|-- THIS SOFTWARE IS PROVIDED BY FREESCALE "AS IS" AND ANY EXPRESSED OR
|-- IMPLIED WARRANTIES, INCLUDING, BUT NOT LIMITED TO, THE IMPLIED WARRANTIES
|-- OF MERCHANTABILITY AND FITNESS FOR A PARTICULAR PURPOSE ARE DISCLAIMED.
|-- IN NO EVENT SHALL FREESCALE OR ITS CONTRIBUTORS BE LIABLE FOR ANY DIRECT,
|-- INDIRECT, INCIDENTAL, SPECIAL, EXEMPLARY, OR CONSEQUENTIAL DAMAGES
|-- (INCLUDING, BUT NOT LIMITED TO, PROCUREMENT OF SUBSTITUTE GOODS OR
|-- SERVICES; LOSS OF USE, DATA, OR PROFITS; OR BUSINESS INTERRUPTION)
|-- HOWEVER CAUSED AND ON ANY THEORY OF LIABILITY, WHETHER IN CONTRACT,
|-- STRICT LIABILITY, OR TORT (INCLUDING NEGLIGENCE OR OTHERWISE) ARISING
|-- IN ANY WAY OUT OF THE USE OF THIS SOFTWARE, EVEN IF ADVISED OF
|-- THE POSSIBILITY OF SUCH DAMAGE.
[IBIS Ver]   5.0
[Comment Char] |_char
[File name]   k10_120_144lqfp_full.ibs
[File Rev]   1.2
[Date]   12/03/2013
[Source]   Freescale, MSG, MCD, Design
[Notes]   IBIS model for K10 microprocessor covers 1.71 - 3.6V range
[Disclaimer]   The model given below represents 144LQFP package on K10 family
[Copyright]   Copyright, Freescale, Inc., 2013
|  Component K10
[Component]   K10
[Manufacturer]  Freescale, Inc.
[Package]
|   typ   min   max
R_pkg   0.13889   0.089996   0.16304
L_pkg   6.188e-9   4.6e-9   7.753e-9
C_pkg   1.406e-12   1.199e-12   1.711e-12
[Pin]   Signal_name   model_name   R_pin   L_pin   C_pin
31   VDDA   POWER
5   VDD   POWER
16   VDD   POWER
43   VDD   POWER
56   VDD   POWER
70   VDD   POWER
94   VDD   POWER
108   VDD   POWER
122   VDD   POWER
135   VDD   POWER
42   VBAT   POWER
36   ADC0SE16   NC   0.14814   6.799e-9   1.29e-12
35   ADC1SE16   NC   0.15075   5.874e-9   1.605e-12
38   DAC0OUT   NC   0.1439   7.173e-9   1.633e-12
39   DAC1OUT   NC   0.14181   7.031e-9   1.609e-12
41   EXTAL32   NC   0.15225   6.57e-9   1.571e-12
28   PGA0DM   NC   0.12556   5.957e-9   1.439e-12
27   PGA0DP   NC   0.12328   5.956e-9   1.323e-12
30   PGA1DM   NC   0.13896   5.302e-9   1.498e-12
29   PGA1DP   NC   0.12975   5.793e-9   1.428e-12
24   PGA2DM   NC   0.12612   5.426e-9   1.253e-12
23   PGA2DP   NC   0.13132   5.164e-9   1.242e-12
26   PGA3DM   NC   0.12285   5.882e-9   1.338e-12
25   PGA3DP   NC   0.12278   5.637e-9   1.298e-12
50   PTA0   io_5vtol   0.14278   6.159e-9   1.422e-12
51   PTA1   io_5vtol   0.14286   6.108e-9   1.337e-12
52   PTA2   io_5vtol   0.14332   5.98e-9   1.337e-12
53   PTA3   io_5vtol   0.14456   5.799e-9   1.346e-12
54   PTA4   io_5vtol   0.14764   5.555e-9   1.299e-12
55   PTA5   io_5vtol   0.1539   5.005e-9   1.264e-12
58   PTA6   io_fast_5vtol  0.14954   5.263e-9   1.291e-12
59   PTA7   io_fast_5vtol  0.14483   5.816e-9   1.336e-12
60   PTA8   io_fast_5vtol  0.14374   6.082e-9   1.385e-12
61   PTA9   io_fast_5vtol  0.1435   6.256e-9   1.329e-12
62   PTA10   io_fast_5vtol  0.14504   6.55e-9   1.37e-12
63   PTA11   io_fast_5vtol  0.14604   6.721e-9   1.362e-12
64   PTA12   io_fast_5vtol  0.14817   6.838e-9   1.393e-12
65   PTA13   io_fast_5vtol  0.15098   6.974e-9   1.475e-12
66   PTA14   io_fast_5vtol  0.15439   7.067e-9   1.507e-12
67   PTA15   io_fast_5vtol  0.1589   7.1e-9   1.585e-12
68   PTA16   io_fast_5vtol  0.15577   6.721e-9   1.564e-12
69   PTA17   io_fast_5vtol  0.16419   6.271e-9   1.534e-12
72   PTA18   io_5vtol   0.16205   6.44e-9   1.293e-12
73   PTA19   io_5vtol   0.15246   7.525e-9   1.292e-12
75   PTA24   io_fast_5vtol  0.14705   7.251e-9   1.711e-12
76   PTA25   io_fast_5vtol  0.14202   7.111e-9   1.574e-12
77   PTA26   io_fast_5vtol  0.13768   6.963e-9   1.55e-12
78   PTA27   io_fast_5vtol  0.13385   6.813e-9   1.519e-12
79   PTA28   io_fast_5vtol  0.13044   6.629e-9   1.413e-12
80   PTA29   io_fast_5vtol  0.12785   6.516e-9   1.437e-12
81   PTB0   io_5vtol   0.12934   6.478e-9   1.329e-12
82   PTB1   io_5vtol   0.12678   6.332e-9   1.37e-12
83   PTB2   io_5vtol   0.12544   6.284e-9   1.394e-12
84   PTB3   io_5vtol   0.12339   6.065e-9   1.249e-12
85   PTB4   io_5vtol   0.12238   5.954e-9   1.26e-12
86   PTB5   io_5vtol   0.12176   5.806e-9   1.298e-12
87   PTB6   io_5vtol   0.12189   5.734e-9   1.29e-12
88   PTB7   io_5vtol   0.12236   5.627e-9   1.342e-12
89   PTB8   io_5vtol   0.12359   5.523e-9   1.305e-12
90   PTB9   io_5vtol   0.12579   5.377e-9   1.238e-12
91   PTB10   io_5vtol   0.12906   5.15e-9   1.278e-12
92   PTB11   io_5vtol   0.13573   4.6e-9   1.242e-12
95   PTB16   io_5vtol   0.13029   4.886e-9   1.199e-12
96   PTB17   io_5vtol   0.12755   5.429e-9   1.322e-12
97   PTB18   io_5vtol   0.12784   5.737e-9   1.313e-12
98   PTB19   io_5vtol   0.1267   6.027e-9   1.37e-12
99   PTB20   io_5vtol   0.12858   6.208e-9   1.359e-12
100   PTB21   io_5vtol   0.12421   6.241e-9   1.419e-12
101   PTB22   io_5vtol   0.12648   6.392e-9   1.422e-12
102   PTB23   io_5vtol   0.12927   6.504e-9   1.503e-12
103   PTC0   io_5vtol   0.13297   6.607e-9   1.602e-12
104   PTC1   io_5vtol   0.1375   6.627e-9   1.536e-12
105   PTC2   io_5vtol   0.14401   6.506e-9   1.577e-12
106   PTC3   io_5vtol   0.15452   5.98e-9   1.59e-12
109   PTC4   io_5vtol   0.15191   7.275e-9   1.253e-12
110   PTC5   io_5vtol   0.14762   7.211e-9   1.535e-12
111   PTC6   io_5vtol   0.14439   7.113e-9   1.542e-12
112   PTC7   io_5vtol   0.14253   7.08e-9   1.527e-12
113   PTC8   io_5vtol   0.14011   6.886e-9   1.414e-12
114   PTC9   io_5vtol   0.13988   6.924e-9   1.489e-12
115   PTC10   io_5vtol   0.13903   6.796e-9   1.48e-12
116   PTC11   io_5vtol   0.14399   6.78e-9   1.353e-12
117   PTC12   io_5vtol   0.14328   6.589e-9   1.442e-12
118   PTC13   io_5vtol   0.1433   6.308e-9   1.363e-12
119   PTC14   io_5vtol   0.14522   6.04e-9   1.387e-12
120   PTC15   io_5vtol   0.15252   5.309e-9   1.347e-12
123   PTC16   io_5vtol   0.15245   5.32e-9   1.261e-12
124   PTC17   io_5vtol   0.14692   5.762e-9   1.317e-12
125   PTC18   io_5vtol   0.14506   5.937e-9   1.38e-12
126   PTC19   io_5vtol   0.14439   6.01e-9   1.303e-12
127   PTD0   io_5vtol   0.14383   6.074e-9   1.304e-12
128   PTD1   io_5vtol   0.1432   6.11e-9   1.332e-12
129   PTD2   io_5vtol   0.14304   6.098e-9   1.298e-12
130   PTD3   io_5vtol   0.14369   6.113e-9   1.374e-12
131   PTD4   io_5vtol   0.14485   6.055e-9   1.311e-12
132   PTD5   io_5vtol   0.14745   5.946e-9   1.34e-12
133   PTD6   io_5vtol   0.15299   5.562e-9   1.278e-12
136   PTD7   io_5vtol   0.094519   5.239e-9   1.36e-12
137   PTD8   io_5vtol   0.14944   6.47e-9   1.472e-12
138   PTD9   io_5vtol   0.1483   6.789e-9   1.563e-12
139   PTD10   io_5vtol   0.14911   7.035e-9   1.591e-12
140   PTD11   io_5vtol   0.15067   7.248e-9   1.566e-12
141   PTD12   io_5vtol   0.14434   7.223e-9   1.472e-12
142   PTD13   io_5vtol   0.14611   7.405e-9   1.666e-12
143   PTD14   io_5vtol   0.14849   7.501e-9   1.697e-12
144   PTD15   io_5vtol   0.15161   7.753e-9   1.354e-12
1   PTE0   io_5vtol   0.14437   7.313e-9   1.274e-12
2   PTE1   io_5vtol   0.1405   6.872e-9   1.603e-12
3   PTE2   io_5vtol   0.1391   6.404e-9   1.665e-12
4   PTE3   io_5vtol   0.14252   5.507e-9   1.561e-12
7   PTE4   io_5vtol   0.14146   5.532e-9   1.372e-12
8   PTE5   io_5vtol   0.13329   5.985e-9   1.41e-12
9   PTE6   io_5vtol   0.12925   6.107e-9   1.373e-12
10   PTE7   io_5vtol   0.12933   6.152e-9   1.393e-12
11   PTE8   io_5vtol   0.12733   5.977e-9   1.362e-12
12   PTE9   io_5vtol   0.12519   5.767e-9   1.221e-12
13   PTE10   io_5vtol   0.1248   5.579e-9   1.305e-12
14   PTE11   io_5vtol   0.12553   5.312e-9   1.334e-12
15   PTE12   io_5vtol   0.12959   4.827e-9   1.279e-12
18   PTE16   io_5vtol   0.1317   4.707e-9   1.231e-12
19   PTE17   io_5vtol   0.12905   5.096e-9   1.211e-12
20   PTE18   io_5vtol   0.13066   5.135e-9   1.351e-12
21   PTE19   io_5vtol   0.13686   4.931e-9   1.245e-12
45   PTE24   io_5vtol   0.16304   5.553e-9   1.491e-12
46   PTE25   io_5vtol   0.1534   6.1e-9   1.395e-12
47   PTE26   io_5vtol   0.14854   6.242e-9   1.399e-12
48   PTE27   io_5vtol   0.14561   6.273e-9   1.355e-12
49   PTE28   io_5vtol   0.14378   6.23e-9   1.351e-12
74   RESETB   io_5vtol   0.089996   6.803e-9   1.672e-12
32   VREFH   NC   0.1438   5.273e-9   1.46e-12
33   VREFL   NC   0.14654   5.492e-9   1.505e-12
37   VREFOUT   NC   0.14765   7.413e-9   1.272e-12
40   XTAL32   NC   0.15245   7.011e-9   1.649e-12
34   VSSA   GND
6   VSS   GND
17   VSS   GND
22   VSS   GND
44   VSS   GND
57   VSS   GND
71   VSS   GND
93   VSS   GND
107   VSS   GND
121   VSS   GND
134   VSS   GND
|End [Component]
[Component] io80u65dgo6m5vtol
|   Component io80u65dgo6m5vtol
| This component was characterised for following simulation conditions:
| Temperature:
|   - Typ: 25.0C,   - Min: 125.0C,   - Max: -40.0C
| External (pad) voltage:
|   - Typ: 3.3V,   - Min: 1.71V,   - Max: 3.6V
| Internal (core) voltage:
|   - Typ: 1.2V,   - Min: 1.08V,   - Max: 1.32V
[Manufacturer] Freescale Semiconductor
[Package]
| variable   typ   min   max
R_pkg   0.2240   0.2240   0.2240
L_pkg   8.5100nH   8.5100nH   8.5100nH
C_pkg   0.2740pF   0.2740pF   0.2740pF
[Pin]  signal_name   model_name   R_pin   L_pin   C_pin
fpad   pad   io_fast_5vtol
pad   pad   io_5vtol
|vsslv vsslv   iGND
|vddlv vddlv   iPOWER
vdd3v  vdd3v   POWER
vss3v  vss3v   GND
|obe   obe   dummy
|do   do   dummy
[Model Selector] io_fast_5vtol
io_fast_5vtol_dse1_sre0   fast io, full drive mode without slew rate
io_fast_5vtol_dse1_sre1   fast io, full drive mode with slew rate
io_fast_5vtol_dse0_sre0   fast io, low drive mode without slew rate
io_fast_5vtol_dse0_sre1   fast io, low drive mode with slew rate
[Model Selector] io_5vtol
io_5vtol_dse1_sre0   io, full drive mode without slew rate
io_5vtol_dse1_sre1   io, full drive mode with slew rate
io_5vtol_dse0_sre0   io, low drive mode without slew rate
io_5vtol_dse0_sre1   io, low drive mode with slew rate
| Models and submodels in the file (8): io_fast_5vtol_dse1_sre0 (I/O), io_5vtol_dse1_sre0 (I/O), io_fast_5vtol_dse1_sre1 (I/O), io_5vtol_dse1_sre1 (I/O), io_fast_5vtol_dse0_sre0 (I/O), io_5vtol_dse0_sre0 (I/O), io_fast_5vtol_dse0_sre1 (I/O), io_5vtol_dse0_sre1 (I/O)
